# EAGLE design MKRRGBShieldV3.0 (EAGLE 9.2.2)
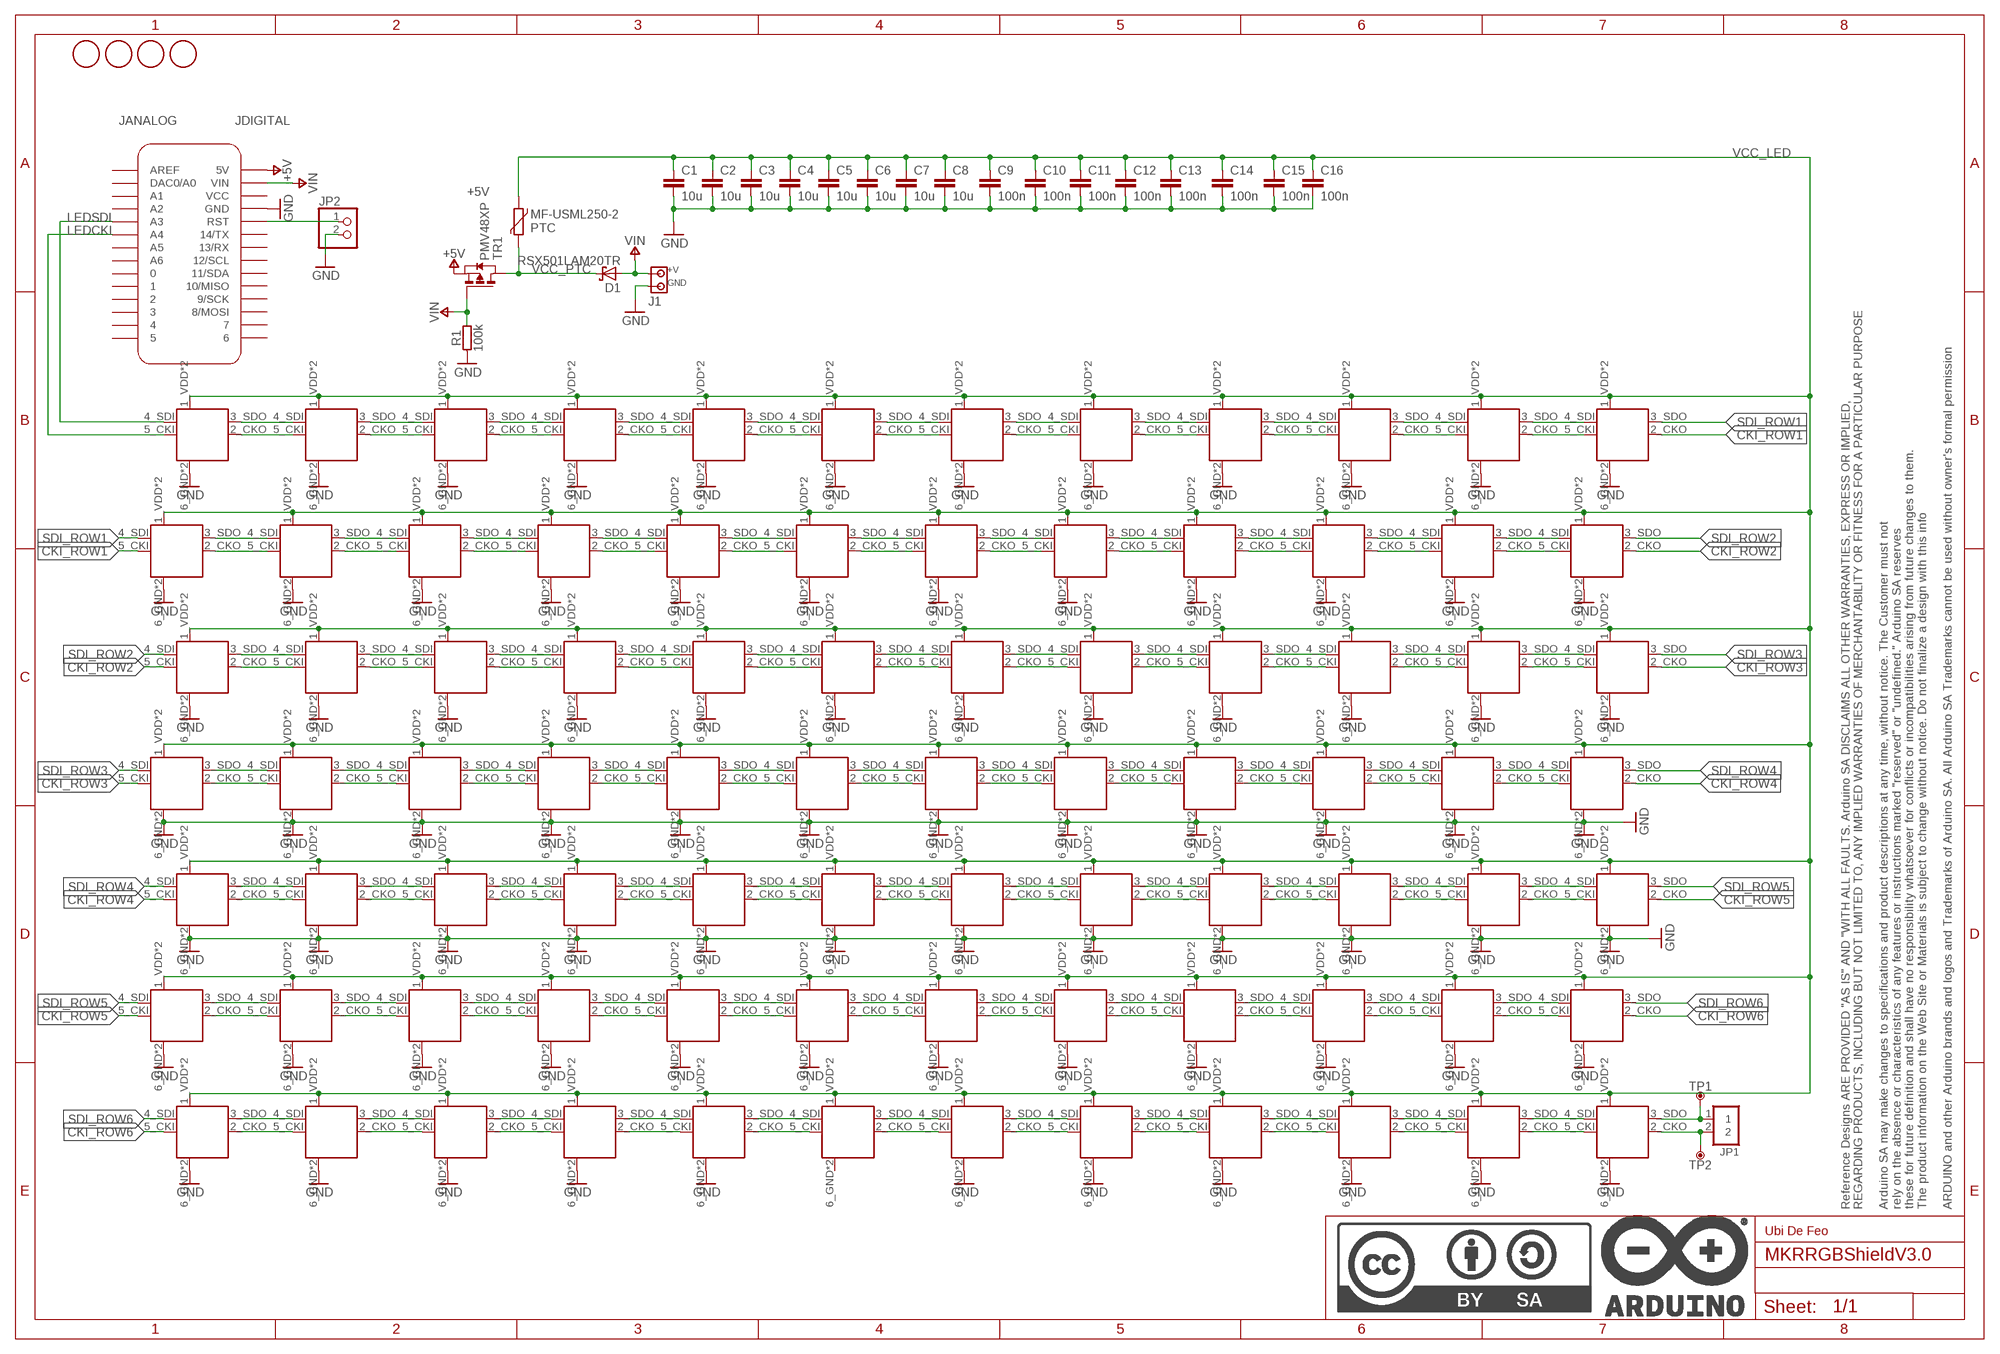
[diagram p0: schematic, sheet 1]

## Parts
32  APA1022020-2018  [APA102-2020_2018]
70  APA1022020-2018  [APA102-2020_2018]
C1  10u  C-10UF-0603  [0603-1608X90N]
C2  10u  C-10UF-0603  [0603-1608X90N]
C3  10u  C-10UF-0603  [0603-1608X90N]
C4  10u  C-10UF-0603  [0603-1608X90N]
C5  10u  C-10UF-0603  [0603-1608X90N]
C6  10u  C-10UF-0603  [0603-1608X90N]
C7  10u  C-10UF-0603  [0603-1608X90N]
C8  10u  C-10UF-0603  [0603-1608X90N]
C9  100n  C-100NF-0402  [0402-1005X55N]
C10  100n  C-100NF-0402  [0402-1005X55N]
C11  100n  C-100NF-0402  [0402-1005X55N]
C12  100n  C-100NF-0402  [0402-1005X55N]
C13  100n  C-100NF-0402  [0402-1005X55N]
C14  100n  C-100NF-0402  [0402-1005X55N]
C15  100n  C-100NF-0402  [0402-1005X55N]
C16  100n  C-100NF-0402  [0402-1005X55N]
D1  RSX501LAM20TR  D_SCHOTTKY-RSX501-SMA  [SMA_DO214AC]
DL1  APA1022020-2018  [APA102-2020_2018]
DL2  APA1022020-2018  [APA102-2020_2018]
DL3  APA1022020-2018  [APA102-2020_2018]
DL4  APA1022020-2018  [APA102-2020_2018]
DL5  APA1022020-2018  [APA102-2020_2018]
DL6  APA1022020-2018  [APA102-2020_2018]
DL7  APA1022020-2018  [APA102-2020_2018]
DL8  APA1022020-2018  [APA102-2020_2018]
DL9  APA1022020-2018  [APA102-2020_2018]
DL10  APA1022020-2018  [APA102-2020_2018]
DL11  APA1022020-2018  [APA102-2020_2018]
DL12  APA1022020-2018  [APA102-2020_2018]
DL13  APA1022020-2018  [APA102-2020_2018]
DL14  APA1022020-2018  [APA102-2020_2018]
DL15  APA1022020-2018  [APA102-2020_2018]
DL16  APA1022020-2018  [APA102-2020_2018]
DL17  APA1022020-2018  [APA102-2020_2018]
DL18  APA1022020-2018  [APA102-2020_2018]
DL19  APA1022020-2018  [APA102-2020_2018]
DL20  APA1022020-2018  [APA102-2020_2018]
DL21  APA1022020-2018  [APA102-2020_2018]
DL22  APA1022020-2018  [APA102-2020_2018]
DL23  APA1022020-2018  [APA102-2020_2018]
DL24  APA1022020-2018  [APA102-2020_2018]
DL25  APA1022020-2018  [APA102-2020_2018]
DL26  APA1022020-2018  [APA102-2020_2018]
DL28  APA1022020-2018  [APA102-2020_2018]
DL29  APA1022020-2018  [APA102-2020_2018]
DL30  APA1022020-2018  [APA102-2020_2018]
DL31  APA1022020-2018  [APA102-2020_2018]
DL33  APA1022020-2018  [APA102-2020_2018]
DL34  APA1022020-2018  [APA102-2020_2018]
DL35  APA1022020-2018  [APA102-2020_2018]
DL36  APA1022020-2018  [APA102-2020_2018]
DL37  APA1022020-2018  [APA102-2020_2018]
DL38  APA1022020-2018  [APA102-2020_2018]
DL39  APA1022020-2018  [APA102-2020_2018]
DL40  APA1022020-2018  [APA102-2020_2018]
DL41  APA1022020-2018  [APA102-2020_2018]
DL42  APA1022020-2018  [APA102-2020_2018]
DL43  APA1022020-2018  [APA102-2020_2018]
DL44  APA1022020-2018  [APA102-2020_2018]
DL45  APA1022020-2018  [APA102-2020_2018]
DL46  APA1022020-2018  [APA102-2020_2018]
DL47  APA1022020-2018  [APA102-2020_2018]
DL48  APA1022020-2018  [APA102-2020_2018]
DL49  APA1022020-2018  [APA102-2020_2018]
DL50  APA1022020-2018  [APA102-2020_2018]
DL51  APA1022020-2018  [APA102-2020_2018]
DL52  APA1022020-2018  [APA102-2020_2018]
DL53  APA1022020-2018  [APA102-2020_2018]
DL54  APA1022020-2018  [APA102-2020_2018]
DL55  APA1022020-2018  [APA102-2020_2018]
DL56  APA1022020-2018  [APA102-2020_2018]
DL57  APA1022020-2018  [APA102-2020_2018]
DL58  APA1022020-2018  [APA102-2020_2018]
DL59  APA1022020-2018  [APA102-2020_2018]
DL60  APA1022020-2018  [APA102-2020_2018]
DL61  APA1022020-2018  [APA102-2020_2018]
DL62  APA1022020-2018  [APA102-2020_2018]
DL63  APA1022020-2018  [APA102-2020_2018]
DL64  APA1022020-2018  [APA102-2020_2018]
DL65  APA1022020-2018  [APA102-2020_2018]
DL66  APA1022020-2018  [APA102-2020_2018]
DL67  APA1022020-2018  [APA102-2020_2018]
DL68  APA1022020-2018  [APA102-2020_2018]
DL69  APA1022020-2018  [APA102-2020_2018]
DL71  APA1022020-2018  [APA102-2020_2018]
DL72  APA1022020-2018  [APA102-2020_2018]
DL73  APA1022020-2018  [APA102-2020_2018]
DL74  APA1022020-2018  [APA102-2020_2018]
DL75  APA1022020-2018  [APA102-2020_2018]
DL76  APA1022020-2018  [APA102-2020_2018]
DL77  APA1022020-2018  [APA102-2020_2018]
DL78  APA1022020-2018  [APA102-2020_2018]
DL79  APA1022020-2018  [APA102-2020_2018]
DL80  APA1022020-2018  [APA102-2020_2018]
DL81  APA1022020-2018  [APA102-2020_2018]
DL82  APA1022020-2018  [APA102-2020_2018]
DL83  APA1022020-2018  [APA102-2020_2018]
DL84  APA1022020-2018  [APA102-2020_2018]
FD1  DNP  FIDUCIAL-1.5MM  [FD-1-1.5]
FD2  DNP  FIDUCIAL-1.5MM  [FD-1-1.5]
FD3  DNP  FIDUCIAL-1.5MM  [FD-1-1.5]
FD4  DNP  FIDUCIAL-1.5MM  [FD-1-1.5]
FRAME1  DNP  A3-FRAME  [FRAME]
J1  -  SCREW2X2.54  [SCREW2]
JANALOG  -  PINHD-1X14-SMD-MKRRGB  [PINHD-DUMMY-1X14-MKRRGB]
JDIGITAL  -  PINHD-1X14-SMD-MKRRGB  [PINHD-DUMMY-1X14-MKRRGB]
JP1  1X02  [1X02]
JP2  PINHD-1X2  [1X02]
MKR1  DNP  MKRBOARD-SMDPIN  [MKRBOARD-SMD-PIN]
PTC  MF-USML250-2  PPTC-MF-USML250-2  [PPTC-1210]
R1  100k  R-100K-0402  [0402-1005X55N]
TP1  DNP  TPTP-1.27MM  [TP-1.27MM]
TP2  DNP  TPTP-1.27MM  [TP-1.27MM]
TR1  PMV48XP  [SOT-23]
U$29  APA1022020-2018  [APA102-2020_2018]

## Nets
+5V: MKR1.5V TR1.2(S)
CKI_ROW1: DL12.2_CKO(CKO) DL13.5_CKI(CKI)
CKI_ROW2: DL24.2_CKO(CKO) DL25.5_CKI(CKI)
CKI_ROW3: DL36.2_CKO(CKO) DL37.5_CKI(CKI)
CKI_ROW4: DL48.2_CKO(CKO) DL49.5_CKI(CKI)
CKI_ROW5: DL60.2_CKO(CKO) DL61.5_CKI(CKI)
CKI_ROW6: DL72.2_CKO(CKO) DL73.5_CKI(CKI)
CKO: DL84.2_CKO(CKO) JP1.2 TP2.X
CKO0: DL1.2_CKO(CKO) DL2.5_CKI(CKI)
DL27: DL28.5_CKI(CKI) U$29.2_CKO(CKO)
GND: 32.6_GND(GND) 32.GNDPAD(GND) 70.6_GND(GND) 70.GNDPAD(GND) C1.2 C2.2 C3.2 C4.2 C5.2 C6.2 C7.2 C8.2 C9.2 C10.2 C11.2 C12.2 C13.2 C14.2 C15.2 C16.2 DL1.6_GND(GND) DL1.GNDPAD(GND) DL2.6_GND(GND) DL2.GNDPAD(GND) DL3.6_GND(GND) DL3.GNDPAD(GND) DL4.6_GND(GND) DL4.GNDPAD(GND) DL5.6_GND(GND) DL5.GNDPAD(GND) DL6.6_GND(GND) DL6.GNDPAD(GND) DL7.6_GND(GND) DL7.GNDPAD(GND) DL8.6_GND(GND) DL8.GNDPAD(GND) DL9.6_GND(GND) DL9.GNDPAD(GND) DL10.6_GND(GND) DL10.GNDPAD(GND) DL11.6_GND(GND) DL11.GNDPAD(GND) DL12.6_GND(GND) DL12.GNDPAD(GND) DL13.6_GND(GND) DL13.GNDPAD(GND) DL14.6_GND(GND) DL14.GNDPAD(GND) DL15.6_GND(GND) DL15.GNDPAD(GND) DL16.6_GND(GND) DL16.GNDPAD(GND) DL17.6_GND(GND) DL17.GNDPAD(GND) DL18.6_GND(GND) DL18.GNDPAD(GND) DL19.6_GND(GND) DL19.GNDPAD(GND) DL20.6_GND(GND) DL20.GNDPAD(GND) DL21.6_GND(GND) DL21.GNDPAD(GND) DL22.6_GND(GND) DL22.GNDPAD(GND) DL23.6_GND(GND) DL23.GNDPAD(GND) DL24.6_GND(GND) DL24.GNDPAD(GND) DL25.6_GND(GND) DL25.GNDPAD(GND) DL26.6_GND(GND) DL26.GNDPAD(GND) DL28.6_GND(GND) DL28.GNDPAD(GND) DL29.6_GND(GND) DL29.GNDPAD(GND) DL30.6_GND(GND) DL30.GNDPAD(GND) DL31.6_GND(GND) DL31.GNDPAD(GND) DL33.6_GND(GND) DL33.GNDPAD(GND) DL34.6_GND(GND) DL34.GNDPAD(GND) DL35.6_GND(GND) DL35.GNDPAD(GND) DL36.6_GND(GND) DL36.GNDPAD(GND) DL37.6_GND(GND) DL37.GNDPAD(GND) DL38.6_GND(GND) DL38.GNDPAD(GND) DL39.6_GND(GND) DL39.GNDPAD(GND) DL40.6_GND(GND) DL40.GNDPAD(GND) DL41.6_GND(GND) DL41.GNDPAD(GND) DL42.6_GND(GND) DL42.GNDPAD(GND) DL43.6_GND(GND) DL43.GNDPAD(GND) DL44.6_GND(GND) DL44.GNDPAD(GND) DL45.6_GND(GND) DL45.GNDPAD(GND) DL46.6_GND(GND) DL46.GNDPAD(GND) DL47.6_GND(GND) DL47.GNDPAD(GND) DL48.6_GND(GND) DL48.GNDPAD(GND) DL49.6_GND(GND) DL49.GNDPAD(GND) DL50.6_GND(GND) DL50.GNDPAD(GND) DL51.6_GND(GND) DL51.GNDPAD(GND) DL52.6_GND(GND) DL52.GNDPAD(GND) DL53.6_GND(GND) DL53.GNDPAD(GND) DL54.6_GND(GND) DL54.GNDPAD(GND) DL55.6_GND(GND) DL55.GNDPAD(GND) DL56.6_GND(GND) DL56.GNDPAD(GND) DL57.6_GND(GND) DL57.GNDPAD(GND) DL58.6_GND(GND) DL58.GNDPAD(GND) DL59.6_GND(GND) DL59.GNDPAD(GND) DL60.6_GND(GND) DL60.GNDPAD(GND) DL61.6_GND(GND) DL61.GNDPAD(GND) DL62.6_GND(GND) DL62.GNDPAD(GND) DL63.6_GND(GND) DL63.GNDPAD(GND) DL64.6_GND(GND) DL64.GNDPAD(GND) DL65.6_GND(GND) DL65.GNDPAD(GND) DL66.6_GND(GND) DL66.GNDPAD(GND) DL67.6_GND(GND) DL67.GNDPAD(GND) DL68.6_GND(GND) DL68.GNDPAD(GND) DL69.6_GND(GND) DL69.GNDPAD(GND) DL71.6_GND(GND) DL71.GNDPAD(GND) DL72.6_GND(GND) DL72.GNDPAD(GND) DL73.6_GND(GND) DL73.GNDPAD(GND) DL74.6_GND(GND) DL74.GNDPAD(GND) DL75.6_GND(GND) DL75.GNDPAD(GND) DL76.6_GND(GND) DL76.GNDPAD(GND) DL77.6_GND(GND) DL77.GNDPAD(GND) DL79.6_GND(GND) DL79.GNDPAD(GND) DL80.6_GND(GND) DL80.GNDPAD(GND) DL81.6_GND(GND) DL81.GNDPAD(GND) DL82.6_GND(GND) DL82.GNDPAD(GND) DL83.6_GND(GND) DL83.GNDPAD(GND) DL84.6_GND(GND) DL84.GNDPAD(GND) J1.GND JP2.2 MKR1.GND R1.1 U$29.6_GND(GND) U$29.GNDPAD(GND)
LEDCKI: DL1.5_CKI(CKI) MKR1.A4
LEDSDI: DL1.4_SDI(SDI) MKR1.A3
N$1: DL2.3_SDO(SDO) DL3.4_SDI(SDI)
N$2: DL2.2_CKO(CKO) DL3.5_CKI(CKI)
N$3: DL3.3_SDO(SDO) DL4.4_SDI(SDI)
N$4: DL3.2_CKO(CKO) DL4.5_CKI(CKI)
N$5: DL4.3_SDO(SDO) DL5.4_SDI(SDI)
N$6: DL4.2_CKO(CKO) DL5.5_CKI(CKI)
N$7: DL5.3_SDO(SDO) DL6.4_SDI(SDI)
N$8: DL5.2_CKO(CKO) DL6.5_CKI(CKI)
N$9: DL6.3_SDO(SDO) DL7.4_SDI(SDI)
N$10: DL6.2_CKO(CKO) DL7.5_CKI(CKI)
N$11: DL7.3_SDO(SDO) DL8.4_SDI(SDI)
N$12: DL7.2_CKO(CKO) DL8.5_CKI(CKI)
N$13: DL8.3_SDO(SDO) DL9.4_SDI(SDI)
N$14: DL8.2_CKO(CKO) DL9.5_CKI(CKI)
N$15: DL9.3_SDO(SDO) DL10.4_SDI(SDI)
N$16: DL9.2_CKO(CKO) DL10.5_CKI(CKI)
N$17: DL10.3_SDO(SDO) DL11.4_SDI(SDI)
N$18: DL10.2_CKO(CKO) DL11.5_CKI(CKI)
N$19: DL11.3_SDO(SDO) DL12.4_SDI(SDI)
N$20: DL11.2_CKO(CKO) DL12.5_CKI(CKI)
N$21: DL13.3_SDO(SDO) DL14.4_SDI(SDI)
N$22: DL13.2_CKO(CKO) DL14.5_CKI(CKI)
N$23: DL14.3_SDO(SDO) DL15.4_SDI(SDI)
N$24: DL14.2_CKO(CKO) DL15.5_CKI(CKI)
N$25: DL15.3_SDO(SDO) DL16.4_SDI(SDI)
N$26: DL15.2_CKO(CKO) DL16.5_CKI(CKI)
N$27: DL16.3_SDO(SDO) DL17.4_SDI(SDI)
N$28: DL16.2_CKO(CKO) DL17.5_CKI(CKI)
N$29: DL17.3_SDO(SDO) DL18.4_SDI(SDI)
N$30: DL17.2_CKO(CKO) DL18.5_CKI(CKI)
N$31: DL18.3_SDO(SDO) DL19.4_SDI(SDI)
N$32: DL18.2_CKO(CKO) DL19.5_CKI(CKI)
N$33: DL19.3_SDO(SDO) DL20.4_SDI(SDI)
N$34: DL19.2_CKO(CKO) DL20.5_CKI(CKI)
N$35: DL20.3_SDO(SDO) DL21.4_SDI(SDI)
N$36: DL20.2_CKO(CKO) DL21.5_CKI(CKI)
N$37: DL21.3_SDO(SDO) DL22.4_SDI(SDI)
N$38: DL21.2_CKO(CKO) DL22.5_CKI(CKI)
N$39: DL22.3_SDO(SDO) DL23.4_SDI(SDI)
N$40: DL22.2_CKO(CKO) DL23.5_CKI(CKI)
N$41: DL23.3_SDO(SDO) DL24.4_SDI(SDI)
N$42: DL23.2_CKO(CKO) DL24.5_CKI(CKI)
N$43: DL25.3_SDO(SDO) DL26.4_SDI(SDI)
N$44: DL25.2_CKO(CKO) DL26.5_CKI(CKI)
N$45: DL26.3_SDO(SDO) U$29.4_SDI(SDI)
N$46: DL26.2_CKO(CKO) U$29.5_CKI(CKI)
N$47: DL28.4_SDI(SDI) U$29.3_SDO(SDO)
N$49: DL28.3_SDO(SDO) DL29.4_SDI(SDI)
N$50: DL28.2_CKO(CKO) DL29.5_CKI(CKI)
N$51: DL29.3_SDO(SDO) DL30.4_SDI(SDI)
N$52: DL29.2_CKO(CKO) DL30.5_CKI(CKI)
N$53: DL30.3_SDO(SDO) DL31.4_SDI(SDI)
N$54: DL30.2_CKO(CKO) DL31.5_CKI(CKI)
N$55: 32.4_SDI(SDI) DL31.3_SDO(SDO)
N$56: 32.5_CKI(CKI) DL31.2_CKO(CKO)
N$57: 32.3_SDO(SDO) DL33.4_SDI(SDI)
N$58: 32.2_CKO(CKO) DL33.5_CKI(CKI)
N$59: DL33.3_SDO(SDO) DL34.4_SDI(SDI)
N$60: DL33.2_CKO(CKO) DL34.5_CKI(CKI)
N$61: DL34.3_SDO(SDO) DL35.4_SDI(SDI)
N$62: DL34.2_CKO(CKO) DL35.5_CKI(CKI)
N$63: DL35.3_SDO(SDO) DL36.4_SDI(SDI)
N$64: DL35.2_CKO(CKO) DL36.5_CKI(CKI)
N$65: DL37.3_SDO(SDO) DL38.4_SDI(SDI)
N$66: DL37.2_CKO(CKO) DL38.5_CKI(CKI)
N$67: DL38.3_SDO(SDO) DL39.4_SDI(SDI)
N$68: DL38.2_CKO(CKO) DL39.5_CKI(CKI)
N$69: DL39.3_SDO(SDO) DL40.4_SDI(SDI)
N$70: DL39.2_CKO(CKO) DL40.5_CKI(CKI)
N$71: DL40.3_SDO(SDO) DL41.4_SDI(SDI)
N$72: DL40.2_CKO(CKO) DL41.5_CKI(CKI)
N$73: DL41.3_SDO(SDO) DL42.4_SDI(SDI)
N$74: DL41.2_CKO(CKO) DL42.5_CKI(CKI)
N$75: DL42.3_SDO(SDO) DL43.4_SDI(SDI)
N$76: DL42.2_CKO(CKO) DL43.5_CKI(CKI)
N$77: DL43.3_SDO(SDO) DL44.4_SDI(SDI)
N$78: DL43.2_CKO(CKO) DL44.5_CKI(CKI)
N$79: DL44.3_SDO(SDO) DL45.4_SDI(SDI)
N$80: DL44.2_CKO(CKO) DL45.5_CKI(CKI)
N$81: DL45.3_SDO(SDO) DL46.4_SDI(SDI)
N$82: DL45.2_CKO(CKO) DL46.5_CKI(CKI)
N$83: DL46.3_SDO(SDO) DL47.4_SDI(SDI)
N$84: DL46.2_CKO(CKO) DL47.5_CKI(CKI)
N$85: DL47.3_SDO(SDO) DL48.4_SDI(SDI)
N$86: DL47.2_CKO(CKO) DL48.5_CKI(CKI)
N$87: DL50.3_SDO(SDO) DL51.4_SDI(SDI)
N$88: DL50.2_CKO(CKO) DL51.5_CKI(CKI)
N$89: DL51.3_SDO(SDO) DL52.4_SDI(SDI)
N$90: DL51.2_CKO(CKO) DL52.5_CKI(CKI)
N$91: DL52.3_SDO(SDO) DL53.4_SDI(SDI)
N$92: DL52.2_CKO(CKO) DL53.5_CKI(CKI)
N$93: DL53.3_SDO(SDO) DL54.4_SDI(SDI)
N$94: DL53.2_CKO(CKO) DL54.5_CKI(CKI)
N$95: DL54.3_SDO(SDO) DL55.4_SDI(SDI)
N$96: DL54.2_CKO(CKO) DL55.5_CKI(CKI)
N$97: DL55.3_SDO(SDO) DL56.4_SDI(SDI)
N$98: DL55.2_CKO(CKO) DL56.5_CKI(CKI)
N$99: DL56.3_SDO(SDO) DL57.4_SDI(SDI)
N$100: DL56.2_CKO(CKO) DL57.5_CKI(CKI)
N$101: DL57.3_SDO(SDO) DL58.4_SDI(SDI)
N$102: DL57.2_CKO(CKO) DL58.5_CKI(CKI)
N$103: DL58.3_SDO(SDO) DL59.4_SDI(SDI)
N$104: DL58.2_CKO(CKO) DL59.5_CKI(CKI)
N$105: DL59.3_SDO(SDO) DL60.4_SDI(SDI)
N$106: DL59.2_CKO(CKO) DL60.5_CKI(CKI)
N$107: DL49.3_SDO(SDO) DL50.4_SDI(SDI)
N$108: DL49.2_CKO(CKO) DL50.5_CKI(CKI)
N$109: DL61.3_SDO(SDO) DL62.4_SDI(SDI)
N$110: DL61.2_CKO(CKO) DL62.5_CKI(CKI)
N$111: DL62.3_SDO(SDO) DL63.4_SDI(SDI)
N$112: DL62.2_CKO(CKO) DL63.5_CKI(CKI)
N$113: DL73.3_SDO(SDO) DL74.4_SDI(SDI)
N$114: DL73.2_CKO(CKO) DL74.5_CKI(CKI)
N$115: DL74.3_SDO(SDO) DL75.4_SDI(SDI)
N$116: DL74.2_CKO(CKO) DL75.5_CKI(CKI)
N$117: DL63.3_SDO(SDO) DL64.4_SDI(SDI)
N$118: DL63.2_CKO(CKO) DL64.5_CKI(CKI)
N$119: DL75.3_SDO(SDO) DL76.4_SDI(SDI)
N$120: DL75.2_CKO(CKO) DL76.5_CKI(CKI)
N$121: DL64.3_SDO(SDO) DL65.4_SDI(SDI)
N$122: DL64.2_CKO(CKO) DL65.5_CKI(CKI)
N$123: DL76.3_SDO(SDO) DL77.4_SDI(SDI)
N$124: DL76.2_CKO(CKO) DL77.5_CKI(CKI)
N$125: DL65.3_SDO(SDO) DL66.4_SDI(SDI)
N$126: DL65.2_CKO(CKO) DL66.5_CKI(CKI)
N$127: DL77.3_SDO(SDO) DL78.4_SDI(SDI)
N$128: DL77.2_CKO(CKO) DL78.5_CKI(CKI)
N$129: DL66.3_SDO(SDO) DL67.4_SDI(SDI)
N$130: DL66.2_CKO(CKO) DL67.5_CKI(CKI)
N$131: DL78.3_SDO(SDO) DL79.4_SDI(SDI)
N$132: DL78.2_CKO(CKO) DL79.5_CKI(CKI)
N$133: DL67.3_SDO(SDO) DL68.4_SDI(SDI)
N$134: DL67.2_CKO(CKO) DL68.5_CKI(CKI)
N$135: DL79.3_SDO(SDO) DL80.4_SDI(SDI)
N$136: DL79.2_CKO(CKO) DL80.5_CKI(CKI)
N$137: DL68.3_SDO(SDO) DL69.4_SDI(SDI)
N$138: DL68.2_CKO(CKO) DL69.5_CKI(CKI)
N$139: DL80.3_SDO(SDO) DL81.4_SDI(SDI)
N$140: DL80.2_CKO(CKO) DL81.5_CKI(CKI)
N$141: 70.4_SDI(SDI) DL69.3_SDO(SDO)
N$142: 70.5_CKI(CKI) DL69.2_CKO(CKO)
N$143: DL81.3_SDO(SDO) DL82.4_SDI(SDI)
N$144: DL81.2_CKO(CKO) DL82.5_CKI(CKI)
N$145: 70.3_SDO(SDO) DL71.4_SDI(SDI)
N$146: 70.2_CKO(CKO) DL71.5_CKI(CKI)
N$147: DL82.3_SDO(SDO) DL83.4_SDI(SDI)
N$148: DL82.2_CKO(CKO) DL83.5_CKI(CKI)
N$149: DL71.3_SDO(SDO) DL72.4_SDI(SDI)
N$150: DL71.2_CKO(CKO) DL72.5_CKI(CKI)
N$151: DL83.3_SDO(SDO) DL84.4_SDI(SDI)
N$152: DL83.2_CKO(CKO) DL84.5_CKI(CKI)
RESET: JP2.1 MKR1.RST
SDI_ROW1: DL12.3_SDO(SDO) DL13.4_SDI(SDI)
SDI_ROW2: DL24.3_SDO(SDO) DL25.4_SDI(SDI)
SDI_ROW3: DL36.3_SDO(SDO) DL37.4_SDI(SDI)
SDI_ROW4: DL48.3_SDO(SDO) DL49.4_SDI(SDI)
SDI_ROW5: DL60.3_SDO(SDO) DL61.4_SDI(SDI)
SDI_ROW6: DL72.3_SDO(SDO) DL73.4_SDI(SDI)
SDO: DL84.3_SDO(SDO) JP1.1 TP1.X
SDO0: DL1.3_SDO(SDO) DL2.4_SDI(SDI)
VCC_LED: 32.1_VDD(VCC) 32.VDDPAD(VCC) 70.1_VDD(VCC) 70.VDDPAD(VCC) C1.1 C2.1 C3.1 C4.1 C5.1 C6.1 C7.1 C8.1 C9.1 C10.1 C11.1 C12.1 C13.1 C14.1 C15.1 C16.1 DL1.1_VDD(VCC) DL1.VDDPAD(VCC) DL2.1_VDD(VCC) DL2.VDDPAD(VCC) DL3.1_VDD(VCC) DL3.VDDPAD(VCC) DL4.1_VDD(VCC) DL4.VDDPAD(VCC) DL5.1_VDD(VCC) DL5.VDDPAD(VCC) DL6.1_VDD(VCC) DL6.VDDPAD(VCC) DL7.1_VDD(VCC) DL7.VDDPAD(VCC) DL8.1_VDD(VCC) DL8.VDDPAD(VCC) DL9.1_VDD(VCC) DL9.VDDPAD(VCC) DL10.1_VDD(VCC) DL10.VDDPAD(VCC) DL11.1_VDD(VCC) DL11.VDDPAD(VCC) DL12.1_VDD(VCC) DL12.VDDPAD(VCC) DL13.1_VDD(VCC) DL13.VDDPAD(VCC) DL14.1_VDD(VCC) DL14.VDDPAD(VCC) DL15.1_VDD(VCC) DL15.VDDPAD(VCC) DL16.1_VDD(VCC) DL16.VDDPAD(VCC) DL17.1_VDD(VCC) DL17.VDDPAD(VCC) DL18.1_VDD(VCC) DL18.VDDPAD(VCC) DL19.1_VDD(VCC) DL19.VDDPAD(VCC) DL20.1_VDD(VCC) DL20.VDDPAD(VCC) DL21.1_VDD(VCC) DL21.VDDPAD(VCC) DL22.1_VDD(VCC) DL22.VDDPAD(VCC) DL23.1_VDD(VCC) DL23.VDDPAD(VCC) DL24.1_VDD(VCC) DL24.VDDPAD(VCC) DL25.1_VDD(VCC) DL25.VDDPAD(VCC) DL26.1_VDD(VCC) DL26.VDDPAD(VCC) DL28.1_VDD(VCC) DL28.VDDPAD(VCC) DL29.1_VDD(VCC) DL29.VDDPAD(VCC) DL30.1_VDD(VCC) DL30.VDDPAD(VCC) DL31.1_VDD(VCC) DL31.VDDPAD(VCC) DL33.1_VDD(VCC) DL33.VDDPAD(VCC) DL34.1_VDD(VCC) DL34.VDDPAD(VCC) DL35.1_VDD(VCC) DL35.VDDPAD(VCC) DL36.1_VDD(VCC) DL36.VDDPAD(VCC) DL37.1_VDD(VCC) DL37.VDDPAD(VCC) DL38.1_VDD(VCC) DL38.VDDPAD(VCC) DL39.1_VDD(VCC) DL39.VDDPAD(VCC) DL40.1_VDD(VCC) DL40.VDDPAD(VCC) DL41.1_VDD(VCC) DL41.VDDPAD(VCC) DL42.1_VDD(VCC) DL42.VDDPAD(VCC) DL43.1_VDD(VCC) DL43.VDDPAD(VCC) DL44.1_VDD(VCC) DL44.VDDPAD(VCC) DL45.1_VDD(VCC) DL45.VDDPAD(VCC) DL46.1_VDD(VCC) DL46.VDDPAD(VCC) DL47.1_VDD(VCC) DL47.VDDPAD(VCC) DL48.1_VDD(VCC) DL48.VDDPAD(VCC) DL49.1_VDD(VCC) DL49.VDDPAD(VCC) DL50.1_VDD(VCC) DL50.VDDPAD(VCC) DL51.1_VDD(VCC) DL51.VDDPAD(VCC) DL52.1_VDD(VCC) DL52.VDDPAD(VCC) DL53.1_VDD(VCC) DL53.VDDPAD(VCC) DL54.1_VDD(VCC) DL54.VDDPAD(VCC) DL55.1_VDD(VCC) DL55.VDDPAD(VCC) DL56.1_VDD(VCC) DL56.VDDPAD(VCC) DL57.1_VDD(VCC) DL57.VDDPAD(VCC) DL58.1_VDD(VCC) DL58.VDDPAD(VCC) DL59.1_VDD(VCC) DL59.VDDPAD(VCC) DL60.1_VDD(VCC) DL60.VDDPAD(VCC) DL61.1_VDD(VCC) DL61.VDDPAD(VCC) DL62.1_VDD(VCC) DL62.VDDPAD(VCC) DL63.1_VDD(VCC) DL63.VDDPAD(VCC) DL64.1_VDD(VCC) DL64.VDDPAD(VCC) DL65.1_VDD(VCC) DL65.VDDPAD(VCC) DL66.1_VDD(VCC) DL66.VDDPAD(VCC) DL67.1_VDD(VCC) DL67.VDDPAD(VCC) DL68.1_VDD(VCC) DL68.VDDPAD(VCC) DL69.1_VDD(VCC) DL69.VDDPAD(VCC) DL71.1_VDD(VCC) DL71.VDDPAD(VCC) DL72.1_VDD(VCC) DL72.VDDPAD(VCC) DL73.1_VDD(VCC) DL73.VDDPAD(VCC) DL74.1_VDD(VCC) DL74.VDDPAD(VCC) DL75.1_VDD(VCC) DL75.VDDPAD(VCC) DL76.1_VDD(VCC) DL76.VDDPAD(VCC) DL77.1_VDD(VCC) DL77.VDDPAD(VCC) DL78.1_VDD(VCC) DL78.VDDPAD(VCC) DL79.1_VDD(VCC) DL79.VDDPAD(VCC) DL80.1_VDD(VCC) DL80.VDDPAD(VCC) DL81.1_VDD(VCC) DL81.VDDPAD(VCC) DL82.1_VDD(VCC) DL82.VDDPAD(VCC) DL83.1_VDD(VCC) DL83.VDDPAD(VCC) DL84.1_VDD(VCC) DL84.VDDPAD(VCC) PTC.P$1 U$29.1_VDD(VCC) U$29.VDDPAD(VCC)
VCC_PTC: D1.C PTC.P$2 TR1.1(D)
VIN: D1.A J1.V+ MKR1.VIN R1.2 TR1.3(G)
Unconnected: MKR1.0 MKR1.1 MKR1.2 MKR1.3 MKR1.4 MKR1.5 MKR1.6 MKR1.7 MKR1.8(8/MOSI) MKR1.9(9/SCK) MKR1.10(10/MISO) MKR1.11(11/SDA) MKR1.12(12/SCL) MKR1.13(13/RX) MKR1.14(14/TX) MKR1.A1 MKR1.A2 MKR1.A5 MKR1.A6 MKR1.AREF MKR1.DAC0/A0 MKR1.VCC

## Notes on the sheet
- Ubi De Feo

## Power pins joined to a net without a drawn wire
GND: DL78.6_GND(GND) DL78.GNDPAD(GND)

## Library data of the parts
32 70 DL1-DL26 DL28-DL31 DL33-DL69 DL71-DL84 U$29 = Arduino-diodes:APA102: -; CODE-ARDUINO: A5307
C1-C8 = Arduino-rcl:C: SMD Capacitor; CODE-ARDUINO: 2213; DATASHEET: http://www.murata.com/~/media/webrenewal/support/library/catalog/products/capacitor/mlcc/c02e.pdf; DISTRIBUTOR-LINK: http://www.digikey.com/product-search/en?keywords=490-10728-1-ND; DISTRIBUTOR-PN: 490-10728-1-ND; MANUFACTURER: Murata; MANUFACTURER-PN: GRM188R61C106KAALD; NOTE: -
C9-C16 = Arduino-rcl:C: SMD Capacitor; CODE-ARDUINO: 0132; DATASHEET: http://www.tdk.com/pdf/TDKMLCCCapRange.pdf; DISTRIBUTOR-LINK: http://www.digikey.com/product-detail/en/tdk-corporation/C1005X5R1H104K050BB/445-5942-1-ND/2443982; DISTRIBUTOR-PN: 445-5942-1-ND; MANUFACTURER: TDK; MANUFACTURER-PN: C1005X5R1H104K050BB; NOTE: -
D1 = Arduino-diodes:D_SCHOTTKY: Schottky Diodes; CODE-ARDUINO: A5388; DATASHEET: https://www.rohm.com/datasheet/RSX501LAM20/rsx501lam20tr-e; DISTRIBUTOR-LINK: https://www.digikey.com/product-detail/en/rohm-semiconductor/RSX501LAM20TR/RSX501LAM20TR-ND/7318348; DISTRIBUTOR-PN: RSX501LAM20TR-ND; MANUFACTURER: Rohm; MANUFACTURER-PN: RSX501LAM20TR
FD1-FD4 = Arduino-utility:FIDUCIAL: Fiducial mount; CODE-ARDUINO: DNP; DATASHEET: DNP; DISTRIBUTOR-LINK: DNP; DISTRIBUTOR-PN: DNP; MANUFACTURER: DNP; MANUFACTURER-PN: DNP
FRAME1 = Arduino-utility:A3-FRAME; CODE-ARDUINO: DNP; DATASHEET: DNP; DISTRIBUTOR-LINK: DNP; DISTRIBUTOR-PN: DNP; MANUFACTURER: DNP; MANUFACTURER-PN: DNP; NOTE: DNP
J1 = Arduino-connectors:SCREW2X2.54: 2.45 Screw terminal Block; CODE-ARDUINO: A5401; DATASHEET: http://www.on-shore.com/wp-content/uploads/2015/09/ostvnxxa150.pdf; DISTRIBUTOR-LINK: http://www.digikey.com/product-detail/en/on-shore-technology-inc/OSTVN02A150/ED10561-ND/1588862; DISTRIBUTOR-PN: ED10561-ND; MANUFACTURER: On Shore Technology Inc.; MANUFACTURER-PN: OSTVN02A150
JANALOG JDIGITAL = Arduino-connectors:PINHD-1X14-SMD-MKRRGB: PIN HEADER 1X14 SMD MKRRGB; CODE-ARDUINO: A5476; DATASHEET: -; DISTRIBUTOR-LINK: -; DISTRIBUTOR-PN: -; MANUFACTURER: -; MANUFACTURER-PN: 20TW-489
JP1 = Ai_Connectors:1X02
JP2 = pinhead:PINHD-1X2: PIN HEADER
MKR1 = Arduino-utility:MKRBOARD: MKR board footprint; CODE-ARDUINO: DNP; DATASHEET: DNP; DISTRIBUTOR-LINK: DNP; DISTRIBUTOR-PN: DNP; MANUFACTURER: DNP; MANUFACTURER-PN: DNP
PTC = Arduino-rcl:PPTC-MF-USML250-2: SMD PTC; CODE-ARDUINO: A5352; DATASHEET: https://nl.mouser.com/datasheet/2/54/fusml-1115405.pdf; DISTRIBUTOR-LINK: https://nl.mouser.com/ProductDetail/Bourns/MF-USML250-2?qs=sGAEpiMZZMsgjL4JkW1EEeamwSwzTegDcao9m1Tn2w%252bDqQsyyTArTA==; DISTRIBUTOR-PN: 652-MF-USML250-2; MANUFACTURER: Bourns Inc; MANUFACTURER-PN: MF-USML250-2; NOTE: NO
R1 = Arduino-rcl:R: SMD Resistor; CODE-ARDUINO: 0134; DATASHEET: www.yageo.com.tw/exep/pages/download/literatures/PYu-R_INT-thick_7.pdf; DISTRIBUTOR-LINK: http://www.digikey.com/product-detail/en/yageo/RC0402FR-07100KL/311-100KLRCT-ND/729473; DISTRIBUTOR-PN: 311-100KLRCT-ND; MANUFACTURER: Yageo; MANUFACTURER-PN: RC0402FR-07100KL; NOTE: NO
TP1 TP2 = Arduino-utility:TP: Testpoint; CODE-ARDUINO: DNP; DATASHEET: DNP; DISTRIBUTOR-LINK: DNP; DISTRIBUTOR-PN: DNP; MANUFACTURER: DNP; MANUFACTURER-PN: DNP
TR1 = Arduino-transistors:PMV48XP: 20 V, 3.5 A P-channel Trench MOSFET - PMV48XP; CODE-ARDUINO: 1039; DATASHEET: https://assets.nexperia.com/documents/data-sheet/PMV48XP.pdf; DISTRIBUTOR-LINK: https://www.digikey.com/product-detail/en/nexperia-usa-inc/PMV48XP215/1727-5907-1-ND/2744665; DISTRIBUTOR-PN: 1727-5907-1-ND; MANUFACTURER: Nexperia; MANUFACTURER-PN: PMV48XP,215; PN-ALTERNATIVE: FDN340P; PN-ALTERNATIVE2: IRLML6402TRPBF

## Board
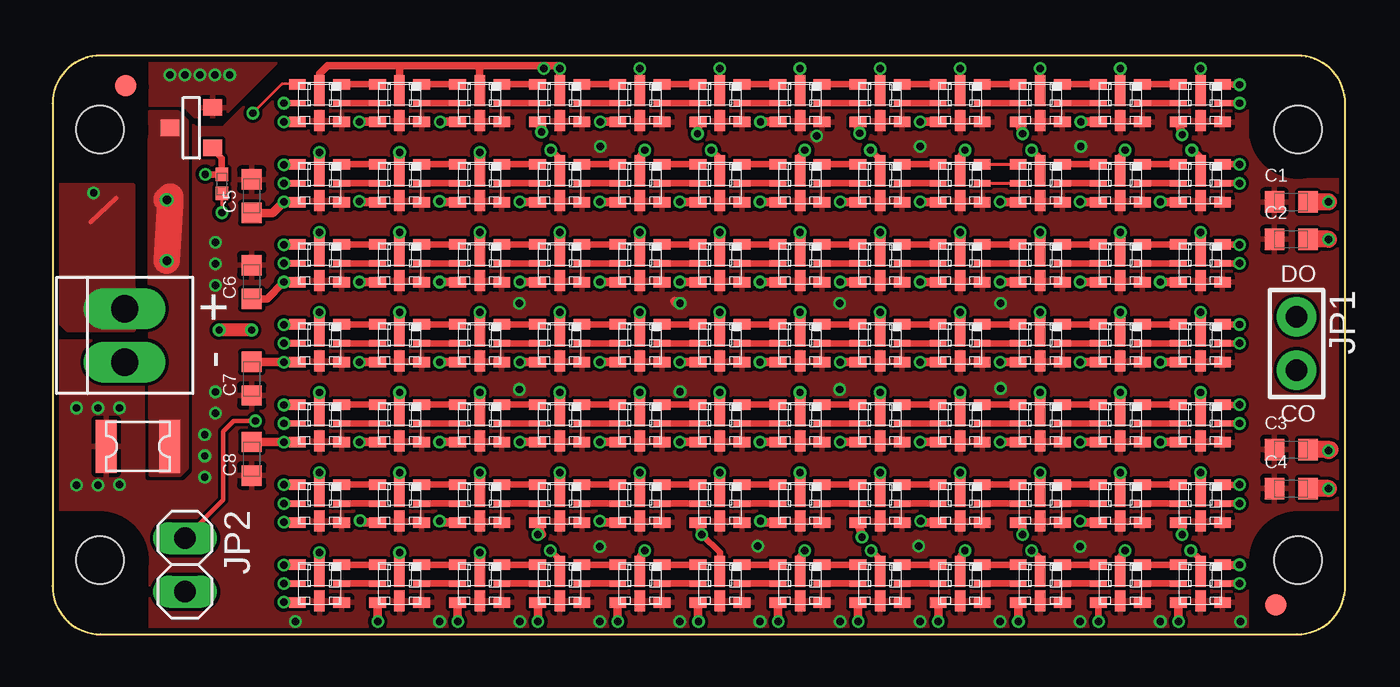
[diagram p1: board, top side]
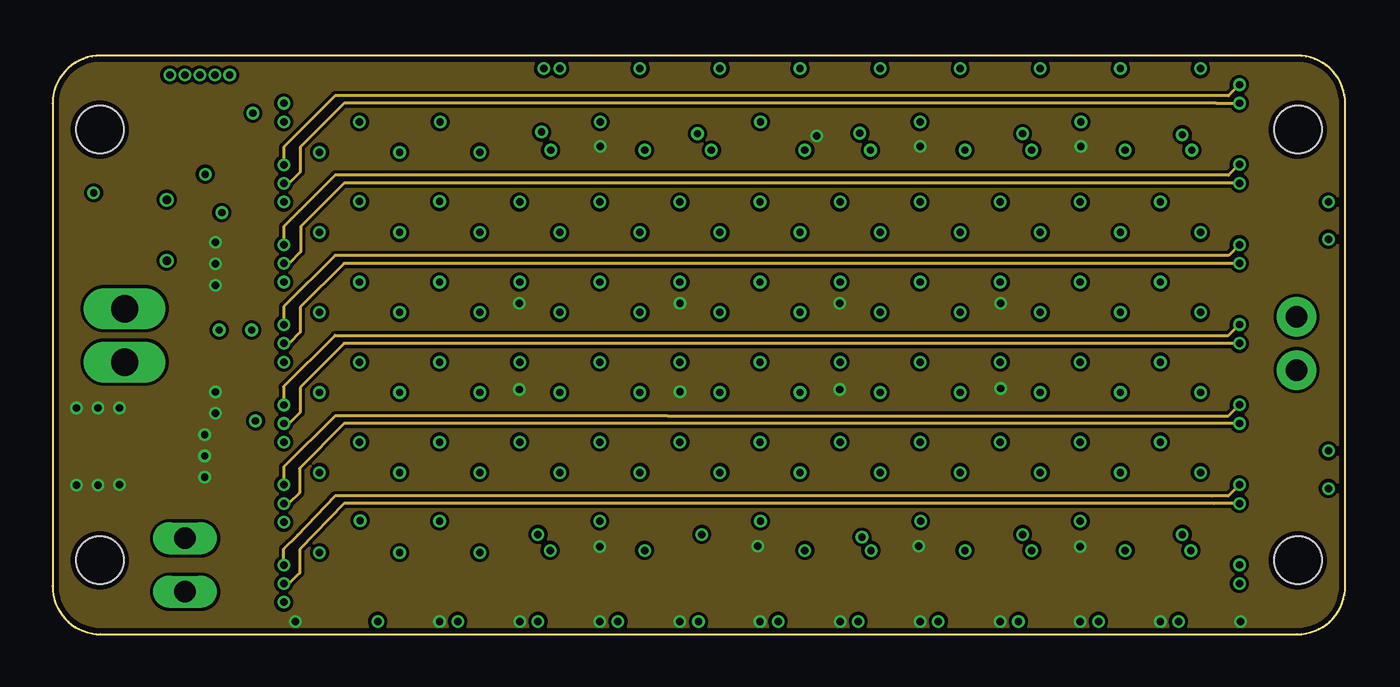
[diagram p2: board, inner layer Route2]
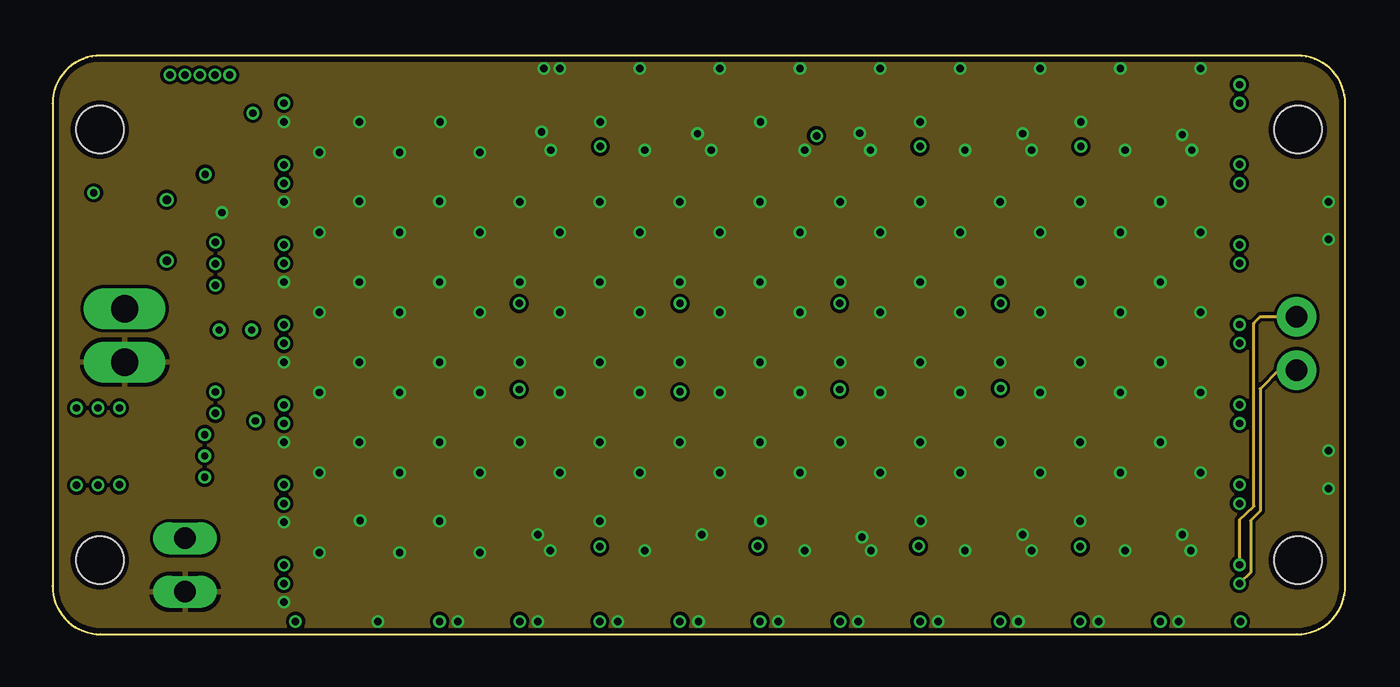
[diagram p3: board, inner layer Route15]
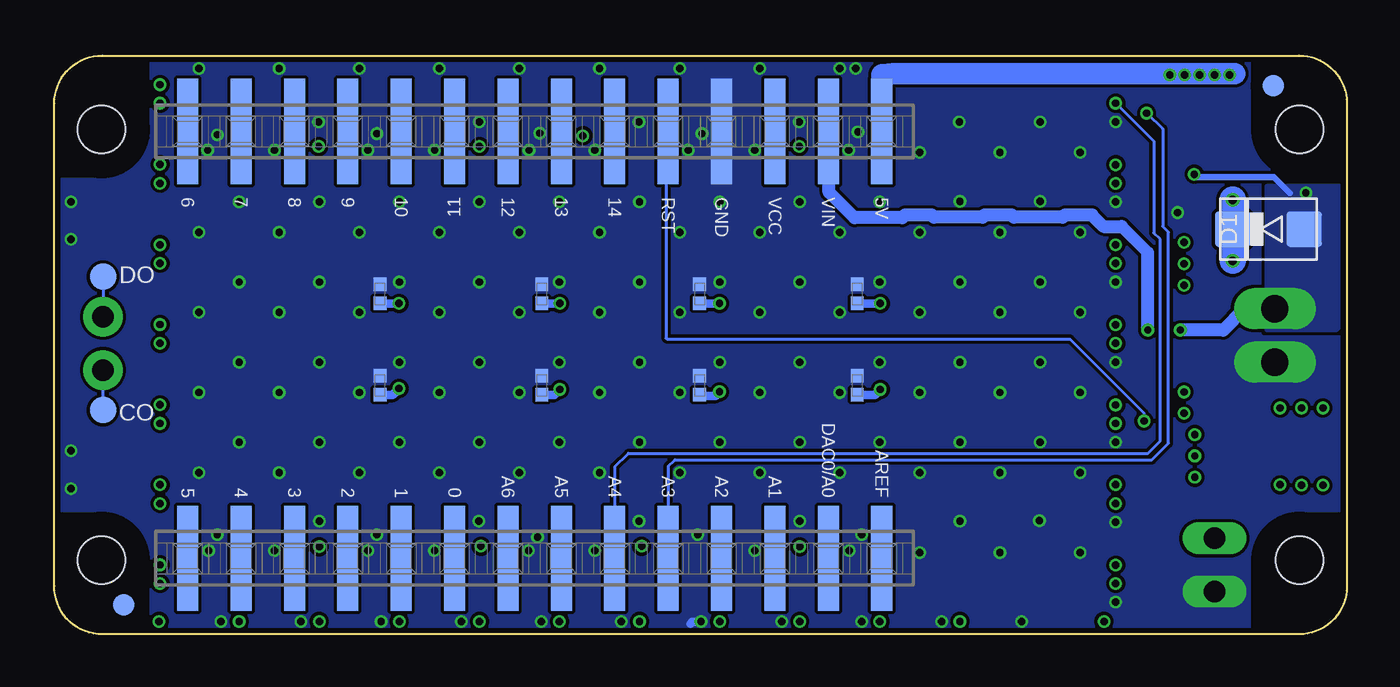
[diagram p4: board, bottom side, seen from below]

Size 61.5 x 27.54 mm. Coordinates in mm from the lower left corner, seen from the top.
Copper layers (1*2*15*16): Top 0.018mm / dielectric 0.36mm / Route2 0.035mm / dielectric 0.71mm / Route15 0.035mm / dielectric 0.2mm / Bottom 0.018mm
Design rules "eC_4Layer_PClass6_BaseCopperO18-I35_eCDefault *": minimum track width 0.15mm, minimum drill 0.35mm, track to track 0.15mm, track to pad 0.15mm, pad to pad 0.15mm, via to via 0.14mm, smd to smd 0mil, copper to edge 0.25mm, drill to drill 0.35mm, minimum pad ring 0.175mm, minimum via ring 0.125mm, stop-mask expansion 0mil, vias tented up to drill 0.45mm, thermal gap 0.2mm

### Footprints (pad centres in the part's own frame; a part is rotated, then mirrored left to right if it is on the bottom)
APA102-2020_2018 = smd 0.8 x 0.5: 1_VDD -1.05,0.9; 3_SDO -1.05,-0.9; 4_SDI 1.05,-0.9; 6_GND 1.05,0.9 | smd 0.8 x 0.3: 2_CKO -1.05,0; 5_CKI 1.05,0 | smd 0.5 x 1.48: GNDPAD 0,-0.59 | smd 0.5 x 1: VDDPAD 0,0.83
0603-1608X90N = smd 0.95 x 1: 1 -0.8,0; 2 0.8,0
0402-1005X55N = smd 0.62 x 0.62: 1 -0.45,0; 2 0.45,0
SMA_DO214AC = smd 1.7 x 1.7: A -1.7,0; C 1.7,0
FD-1-1.5 = smd 1.016 x 1.016: P$1 0,0
SCREW2 = drill 1.3 long: GND 1.27,0; V+ -1.27,0
1X02 = drill 1.016 pad 1.88: 1 -1.27,0; 2 1.27,0
1X02' = drill 1.016 long: 1 -1.27,0; 2 1.27,0
MKRBOARD-SMD-PIN = smd 1 x 5 bottom: 0 42.455,3.61; 1 44.995,3.61; 2 47.535,3.61; 3 50.075,3.61; 4 52.615,3.61; 5 55.155,3.61; 5V 22.135,23.93; 6 55.155,23.93; 7 52.615,23.93; 8 50.075,23.93; 9 47.535,23.93; 10 44.995,23.93; 11 42.455,23.93; 12 39.915,23.93; 13 37.375,23.93; 14 34.835,23.93; A1 27.215,3.61; A2 29.755,3.61; A3 32.295,3.61; A4 34.835,3.61; A5 37.375,3.61; A6 39.915,3.61; AREF 22.135,3.61; DAC0/A0 24.675,3.61; GND 29.755,23.93; RST 32.295,23.93; VCC 27.215,23.93; VIN 24.675,23.93 | hole 2.25: 59.25,3.52; 59.25,24.02; 2.25,3.52; 2.25,24.02
PPTC-1210 = smd 1 x 2.5: P$1 -1.5,0; P$2 1.5,0
TP-1.27MM = smd 1.27 x 1.27 bottom: X 0,0
SOT-23 = smd 0.787 x 0.889: 1 -0.025,1.016; 2 0.94,-1.016; 3 -0.991,-1.016

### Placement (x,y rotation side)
32  39.37,17.65 180 top
70  46.99,6.22 180 top
C1  58.93,20.57 0 top
C2  58.93,18.8 0 top
C3  58.93,8.79 0 top
C4  58.93,6.93 0 top
C5  9.47,20.85 270 top
C6  9.47,16.76 270 top
C7  9.47,12.17 90 top
C8  9.47,8.35 90 top
C9  30.8,16.2 90 bottom
C10  23.3,16.2 90 bottom
C11  38.3,16.2 90 bottom
C12  46,16.2 90 bottom
C13  23.3,11.85 90 bottom
C14  30.8,11.85 90 bottom
C15  38.3,11.85 90 bottom
C16  46,11.85 90 bottom
D1  3.73,19.28 180 bottom
DL1  12.7,25.27 180 top
DL2  16.51,25.27 180 top
DL3  20.32,25.27 180 top
DL4  24.13,25.27 180 top
DL5  27.94,25.27 180 top
DL6  31.75,25.27 180 top
DL7  35.56,25.27 180 top
DL8  39.37,25.27 180 top
DL9  43.18,25.27 180 top
DL10  46.99,25.27 180 top
DL11  50.8,25.27 180 top
DL12  54.61,25.27 180 top
DL13  12.7,21.46 180 top
DL14  16.51,21.46 180 top
DL15  20.32,21.46 180 top
DL16  24.13,21.46 180 top
DL17  27.94,21.46 180 top
DL18  31.75,21.46 180 top
DL19  35.56,21.46 180 top
DL20  39.37,21.46 180 top
DL21  43.18,21.46 180 top
DL22  46.99,21.46 180 top
DL23  50.8,21.46 180 top
DL24  54.61,21.46 180 top
DL25  12.7,17.65 180 top
DL26  16.51,17.65 180 top
DL28  24.13,17.65 180 top
DL29  27.94,17.65 180 top
DL30  31.75,17.65 180 top
DL31  35.56,17.65 180 top
DL33  43.18,17.65 180 top
DL34  46.99,17.65 180 top
DL35  50.8,17.65 180 top
DL36  54.61,17.65 180 top
DL37  12.7,13.84 180 top
DL38  16.51,13.84 180 top
DL39  20.32,13.84 180 top
DL40  24.13,13.84 180 top
DL41  27.94,13.84 180 top
DL42  31.75,13.84 180 top
DL43  35.56,13.84 180 top
DL44  39.37,13.84 180 top
DL45  43.18,13.84 180 top
DL46  46.99,13.84 180 top
DL47  50.8,13.84 180 top
DL48  54.61,13.84 180 top
DL49  12.7,10.03 180 top
DL50  16.51,10.03 180 top
DL51  20.32,10.03 180 top
DL52  24.13,10.03 180 top
DL53  27.94,10.03 180 top
DL54  31.75,10.03 180 top
DL55  35.56,10.03 180 top
DL56  39.37,10.03 180 top
DL57  43.18,10.03 180 top
DL58  46.99,10.03 180 top
DL59  50.8,10.03 180 top
DL60  54.61,10.03 180 top
DL61  12.7,6.22 180 top
DL62  16.51,6.22 180 top
DL63  20.32,6.22 180 top
DL64  24.13,6.22 180 top
DL65  27.94,6.22 180 top
DL66  31.75,6.22 180 top
DL67  35.56,6.22 180 top
DL68  39.37,6.22 180 top
DL69  43.18,6.22 180 top
DL71  50.8,6.22 180 top
DL72  54.61,6.22 180 top
DL73  12.7,2.41 180 top
DL74  16.51,2.41 180 top
DL75  20.32,2.41 180 top
DL76  24.13,2.41 180 top
DL77  27.94,2.41 180 top
DL78  31.75,2.41 180 top
DL79  35.56,2.41 180 top
DL80  39.37,2.41 180 top
DL81  43.18,2.41 180 top
DL82  46.99,2.41 180 top
DL83  50.8,2.41 180 top
DL84  54.61,2.41 180 top
FD1  58.2,1.4 0 bottom
FD2  3.48,26.11 0 top
FD3  3.5,26.1 0 bottom
FD4  58.2,1.4 0 top
FRAME1  0,-1.27 0 top
J1  3.43,14.22 270 top
JANALOG  not placed on the board
JDIGITAL  not placed on the board
JP1  59.18,13.84 270 top
JP2  [1X02']  6.3,3.3 270 top
MKR1  0,0 0 top
PTC  4.06,8.94 0 top
R1  8.05,21.43 90 top
TP1  59.18,17.02 0 top
TP2  59.18,10.67 0 top
TR1  6.6,24.13 90 top
U$29  20.32,17.65 180 top

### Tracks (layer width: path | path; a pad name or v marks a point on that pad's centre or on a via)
+5V  (via drill 0.35)
  Top 0.406: v6.29,26.62 6.35,26.56
  Bottom 0.203: v6.29,26.62 6.29,26.67
  Bottom 1.016: MKR1.5V 22.14,26.63 21.59,26.67 6.29,26.67 5.33,26.67
  other vias: 7.72,26.62 8.43,26.62 5.58,26.62 7.01,26.62
  pour Top (isolate 0.025, rank 5): 4.57,27.43 4.57,25.15 6.22,25.15 6.73,24.64 8.13,24.64 10.92,27.43
  pour Top (no thermals): 4.65,27.18 10.41,27.18 9.4,26.16 4.65,26.16
CKI_ROW1  (via drill 0.35)
  Top 0.305: DL13.5_CKI v11,21.46 | DL12.2_CKO v56.46,25.27
  Route2 0.152: v56.46,25.27 55.37,25.27 13.87,25.27 11.79,23.19 11.79,22 11.25,21.46 v11,21.46
CKI_ROW2  (via drill 0.35)
  Top 0.305: DL25.5_CKI v11,17.65 | DL24.2_CKO v56.46,21.46
  Route2 0.152: v56.46,21.46 13.87,21.46 11.81,19.41 11.81,18.21 11.25,17.65 v11,17.65
CKI_ROW3  (via drill 0.35)
  Top 0.305: v56.46,17.65 DL36.2_CKO | DL37.5_CKI v11,13.84
  Route2 0.152: v56.46,17.65 13.87,17.65 11.79,15.57 11.79,14.38 11.25,13.84 v11,13.84
CKI_ROW4  (via drill 0.35)
  Top 0.305: DL48.2_CKO v56.46,13.84 | DL49.5_CKI v11,10.03
  Route2 0.152: v11,10.03 11.25,10.03 11.79,10.57 11.79,11.74 13.87,13.84 v56.46,13.84
CKI_ROW5  (via drill 0.35)
  Top 0.305: DL61.5_CKI v11,6.22 | DL60.2_CKO v56.46,10.03
  Route2 0.152: v11,6.22 11.23,6.22 11.74,6.73 11.74,7.89 13.87,10.03 v56.46,10.03
CKI_ROW6  (via drill 0.35)
  Top 0.305: DL73.5_CKI v11,2.41 | v56.46,6.22 DL72.2_CKO
  Route2 0.152: v11,2.41 11.25,2.41 11.76,2.92 11.76,4.04 13.87,6.22 55.27,6.22 v56.46,6.22
CKO  (via drill 0.35)
  Top 0.305: DL84.2_CKO v56.46,2.41
  Route15 0.152: v56.46,2.41 56.47,2.41 57,2.94 57,5.41 57.45,5.87 57.45,11.68 58.34,12.57 JP1.2
  Bottom 0.152: TP2.X JP1.2
CKO0
  Top 0.305: DL1.2_CKO DL2.5_CKI
DL27
  Top 0.305: U$29.2_CKO DL28.5_CKI
GND  (via drill 0.35)
  Top 0.152: 23.08,24.4 DL4.6_GND | 30.7,24.4 DL6.6_GND | 38.32,24.4 DL8.6_GND | 45.94,24.4 DL10.6_GND | 53.56,24.4 DL12.6_GND | 45.95,5.36 45.95,5.33 | 34.51,1.54 DL79.6_GND | 11.65,1.54 DL73.6_GND | 53.56,1.54 DL84.6_GND | 30.7,5.35 DL66.6_GND | 38.32,5.35 DL68.6_GND | 11.64,12.96 11.64,12.95 | 15.45,12.96 15.45,12.95 | 19.26,12.96 19.26,12.95 | 23.07,12.96 23.07,12.95 | 26.88,12.96 26.88,12.95 | 30.69,12.96 30.69,12.95 | 34.5,12.96 34.5,12.95 | 38.31,12.96 38.31,12.95 | 42.13,12.97 DL45.6_GND | 45.94,12.97 DL46.6_GND | 49.74,12.96 49.74,12.95 | 53.55,12.96 53.55,12.95 | 15.45,16.77 15.45,16.76 | 19.26,16.77 19.26,16.76 | 23.07,16.77 23.07,16.76 | 34.5,16.77 34.5,16.76 | 42.13,16.78 DL33.6_GND | 45.93,16.77 45.93,16.76 | 49.74,16.77 49.74,16.76 | 11.65,20.59 DL13.6_GND | R1.1 v8.05,20.07 | DL1.GNDPAD 12.7,25.68 | DL68.GNDPAD v39.37,7.7
  Top 0.254: DL8.GNDPAD v39.37,26.92 | DL7.GNDPAD v35.56,26.92 | DL6.GNDPAD v31.75,26.92 | DL5.GNDPAD v27.94,26.92
  Top 0.305: DL12.GNDPAD v54.61,26.92 | DL11.GNDPAD v50.8,26.92 | DL10.GNDPAD v46.99,26.92 | DL9.GNDPAD v43.18,26.92 | DL13.GNDPAD v12.7,22.94 | DL14.GNDPAD v16.51,22.94 | DL15.GNDPAD v20.32,22.94 | DL16.GNDPAD 24.13,22.66 23.75,23.04 v23.7,23.04 | DL17.GNDPAD 27.94,22.78 v28.17,23.04 | DL18.GNDPAD 31.75,22.66 v31.34,23.04 | DL19.GNDPAD 35.56,22.78 v35.79,23.04 | v38.91,23.04 39.37,22.61 DL20.GNDPAD | DL21.GNDPAD 43.18,22.78 v43.41,23.04 | v46.58,23.04 46.99,22.66 DL22.GNDPAD | DL23.GNDPAD 50.8,22.78 v51.03,23.04 | DL25.GNDPAD v12.7,19.13 | DL26.GNDPAD v16.51,19.13 | U$29.GNDPAD v20.32,19.13 | DL28.GNDPAD v24.13,19.13 | DL29.GNDPAD v27.94,19.13 | DL30.GNDPAD v31.75,19.13 | DL31.GNDPAD v35.56,19.13 | 32.GNDPAD v39.37,19.13 | DL33.GNDPAD v43.18,19.13 | DL34.GNDPAD v46.99,19.13 | DL35.GNDPAD v50.8,19.13 | DL36.GNDPAD v54.61,19.13 | DL37.GNDPAD v12.7,15.32 | DL38.GNDPAD v16.51,15.32 | DL39.GNDPAD v20.32,15.32 | DL40.GNDPAD v24.13,15.32 | DL41.GNDPAD v27.94,15.32 | DL42.GNDPAD v31.75,15.32 | DL44.GNDPAD v39.37,15.32 | DL45.GNDPAD v43.18,15.32 | DL46.GNDPAD v46.99,15.32 | DL47.GNDPAD v50.8,15.32 | DL48.GNDPAD v54.61,15.32 | DL43.GNDPAD v35.56,15.32 | DL49.GNDPAD v12.7,11.51 | DL50.GNDPAD v16.51,11.51 | DL53.GNDPAD v27.94,11.51 | DL54.GNDPAD v31.75,11.51 | DL55.GNDPAD v35.56,11.51 | DL56.GNDPAD v39.37,11.51 | DL57.GNDPAD v43.18,11.51 | DL58.GNDPAD v46.99,11.51 | DL59.GNDPAD v50.8,11.51 | DL60.GNDPAD v54.61,11.51 | DL61.GNDPAD v12.7,7.7 | DL62.GNDPAD v16.51,7.7 | DL63.GNDPAD v20.32,7.7 | DL64.GNDPAD v24.13,7.7 | DL65.GNDPAD v27.94,7.7 | DL66.GNDPAD v31.75,7.7 | DL67.GNDPAD v35.56,7.7 | DL69.GNDPAD v43.18,7.7 | 70.GNDPAD v46.99,7.7 | DL71.GNDPAD v50.8,7.7 | DL72.GNDPAD v54.61,7.7
  Top 0.305: v12.7,3.89 DL73.GNDPAD | DL74.GNDPAD v16.51,3.89 | DL75.GNDPAD v20.32,3.89 | DL76.GNDPAD 24.13,3.56 v23.67,3.99 | DL77.GNDPAD 27.94,3.73 v28.17,3.99 | DL79.GNDPAD 35.56,3.73 v35.79,3.99 | DL80.GNDPAD 39.37,3.58 v38.94,3.99 | DL81.GNDPAD 43.18,3.73 v43.41,3.99 | DL82.GNDPAD 46.99,3.61 v46.58,3.99 | DL83.GNDPAD 50.8,3.73 v51.03,3.99 | DL84.GNDPAD 54.61,3.56 v54.15,3.99 | v54.2,23.04 54.3,23.04 54.61,22.73 DL24.GNDPAD | DL51.GNDPAD v20.32,11.51 | DL52.GNDPAD v24.13,11.51 | DL83.6_GND 49.75,0.81 49.76,0.8 v49.76,0.61 | DL13.6_GND 11.01,20.58 v11,20.57 | DL25.6_GND 11.84,16.76 v11,16.76 | DL78.GNDPAD 31.75,3.89 30.9,4.74
  Top 0.356: 12.7,25.68 12.7,26.67 13.08,27.05 16.51,27.05 | 16.51,27.05 20.32,27.05 | DL2.GNDPAD 16.51,27.05 | DL3.GNDPAD 20.32,27.05 | 20.32,27.05 23.37,27.05 | 23.37,27.05 24,27.05 v24.13,26.92 DL4.GNDPAD | v23.37,26.92 23.37,27.05 | v11,16.76 10.2,15.96 C6.2
  Top 0.406: DL84.6_GND 53.57,1.52 v53.57,0.61 | DL73.6_GND 11.64,1.52 v11,1.52 | DL61.6_GND 11.64,5.33 v11,5.33 | 45.95,5.33 70.6_GND 46.15,5.33 v46.15,4.75 | DL60.6_GND 53.55,9.14 v52.7,9.14 | DL59.6_GND 49.74,9.14 v48.9,9.14 | DL58.6_GND 45.93,9.14 v45.09,9.14 | DL57.6_GND 42.12,9.14 v41.27,9.14 | DL56.6_GND 38.31,9.14 v37.47,9.14 | DL55.6_GND 34.5,9.14 v33.66,9.14 | DL54.6_GND 30.69,9.14 v29.84,9.14 | DL53.6_GND 26.88,9.14 v26.04,9.14 | DL52.6_GND 23.07,9.14 v22.23,9.14 | DL51.6_GND 19.26,9.14 v18.41,9.14 | DL50.6_GND 15.45,9.14 v14.61,9.14 | DL49.6_GND 11.64,9.14 v11,9.14 9.67,9.14 C8.2 | DL48.6_GND 53.55,12.95 v52.7,12.95 | DL47.6_GND 49.74,12.95 v48.9,12.95 | DL46.6_GND 45.93,12.95 v45.09,12.95 | DL45.6_GND 42.12,12.95 v41.27,12.95 | DL44.6_GND 38.31,12.95 v37.47,12.95 | DL43.6_GND 34.5,12.95 v33.66,12.95 | DL42.6_GND 30.69,12.95 v29.84,12.95 | DL41.6_GND 26.88,12.95 v26.04,12.95 | DL40.6_GND 23.07,12.95 v22.23,12.95 | DL39.6_GND 19.26,12.95 v18.41,12.95 | DL38.6_GND 15.45,12.95 v14.61,12.95 | DL37.6_GND 11.64,12.95 v11,12.95 9.49,12.95 C7.2 | DL36.6_GND 53.55,16.76 v52.7,16.76 | DL35.6_GND 49.74,16.76 v48.9,16.76 | DL34.6_GND 45.93,16.76 v45.09,16.76 | DL33.6_GND 42.12,16.76 v41.27,16.76 | 32.6_GND 38.31,16.76 v37.47,16.76 | DL31.6_GND 34.5,16.76 v33.66,16.76 | DL30.6_GND 30.69,16.76 v29.84,16.76 | DL29.6_GND 26.88,16.76 v26.04,16.76 | DL28.6_GND 23.07,16.76 v22.23,16.76 | U$29.6_GND 19.26,16.76 v18.41,16.76 | DL26.6_GND 15.45,16.76 v14.61,16.76 | DL14.6_GND 14.62,20.56 v14.61,20.6 | DL15.6_GND 18.43,20.56 v18.41,20.6 | DL16.6_GND v22.24,20.56 v22.23,20.57 | DL17.6_GND v26.05,20.56 v26.04,20.57 | DL18.6_GND 29.86,20.56 v29.84,20.57
  Top 0.406: DL19.6_GND v33.67,20.56 v33.66,20.57 | DL20.6_GND v37.48,20.56 v37.47,20.57 | DL21.6_GND 41.29,20.56 v41.27,20.57 | DL22.6_GND v45.1,20.56 v45.09,20.57 | DL23.6_GND 49.74,20.57 v48.9,20.57 | DL24.6_GND 53.55,20.57 v52.7,20.57 | DL1.6_GND 11.64,24.38 v11,24.38 | v45.95,0.61 DL82.6_GND | v42.14,0.61 DL81.6_GND | v38.33,0.61 DL80.6_GND | v34.52,0.61 34.52,1.53 34.51,1.54 | v23.09,0.61 DL76.6_GND | v19.28,0.61 DL75.6_GND | v15.47,0.61 DL74.6_GND | v26.9,0.61 26.89,0.67 DL77.6_GND | DL62.6_GND 14.72,5.32 v14.63,5.41 | DL68.6_GND v38.52,4.62 v38.51,4.62 | DL66.6_GND 30.9,4.74 v30.89,4.75 | DL64.6_GND 23.28,4.75 v23.09,4.75 | DL63.6_GND 18.48,5.32 v18.41,5.38 | v26.04,5.38 26.1,5.32 DL65.6_GND | v33.68,5.38 33.74,5.32 DL67.6_GND | DL69.6_GND 41.36,5.32 v41.3,5.38 | v48.9,5.38 48.96,5.32 DL71.6_GND | DL4.6_GND 23.28,23.91 v23.27,23.9 | v30.69,23.82 v30.7,23.84 DL6.6_GND | DL8.6_GND 38.32,24.12 38.42,23.86 v38.41,23.85 | v46.15,23.82 v46.14,23.84 DL10.6_GND | v53.75,23.77 53.76,23.79 DL12.6_GND | DL72.6_GND 53.75,5.33 v53.75,4.75 | C5.2 10.47,20.05 v11,20.57 | DL2.6_GND 15.65,24.38 v14.61,24.38 | DL3.6_GND 19.46,24.38 v18.44,24.38 | DL5.6_GND 27.08,24.38 v26.06,24.38 | DL7.6_GND 34.7,24.38 v33.68,24.38 | DL9.6_GND 42.32,24.38 v41.27,24.38 | DL11.6_GND 49.94,24.38 v48.92,24.38 | DL78.6_GND 30.7,0.54 30.73,0.51 v30.73,0.6
  Top 0.813: v60.7,18.8 C2.2 | v60.7,6.93 C4.2 | v60.7,8.73 60.74,8.78 60.77,8.79 C3.2 | v60.7,20.57 C1.2
  Bottom 0.406: v30.73,0.6 31.15,0.6 31.24,0.51
  pour Bottom (rank 6, no thermals): 0,0 0,27.43 61.47,27.43 61.47,0
  pour Route15: 0,0 0,27.5 61.4,27.5 61.4,0
LEDCKI  (via drill 0.35)
  Top 0.305: v11,25.27 DL1.5_CKI
  Bottom 0.152: MKR1.A4 34.84,7.96 34.19,8.61 9.47,8.61 8.89,9.19 8.89,18.8 9.2,19.1 9.2,23.47 v11,25.27
LEDSDI  (via drill 0.35)
  Top 0.152: v9.53,24.8 10.93,26.2 DL1.4_SDI
  Bottom 0.152: MKR1.A3 32.3,7.99 31.98,8.31 9.27,8.31 8.49,9.09 8.49,19.13 8.77,19.41 8.77,24.06 9.51,24.8 v9.53,24.8
N$1
  Top 0.305: DL2.3_SDO DL3.4_SDI
N$2
  Top 0.305: DL2.2_CKO DL3.5_CKI
N$3
  Top 0.305: DL3.3_SDO DL4.4_SDI
N$4
  Top 0.305: DL3.2_CKO DL4.5_CKI
N$5
  Top 0.305: DL4.3_SDO DL5.4_SDI
N$6
  Top 0.305: DL4.2_CKO DL5.5_CKI
N$7
  Top 0.305: DL5.3_SDO DL6.4_SDI
N$8
  Top 0.305: DL5.2_CKO DL6.5_CKI
N$9
  Top 0.305: DL6.3_SDO DL7.4_SDI
N$10
  Top 0.305: DL6.2_CKO DL7.5_CKI
N$11
  Top 0.305: DL7.3_SDO DL8.4_SDI
N$12
  Top 0.305: DL7.2_CKO DL8.5_CKI
N$13
  Top 0.305: DL8.3_SDO DL9.4_SDI
N$14
  Top 0.305: DL8.2_CKO DL9.5_CKI
N$15
  Top 0.305: DL9.3_SDO DL10.4_SDI
N$16
  Top 0.305: DL9.2_CKO DL10.5_CKI
N$17
  Top 0.305: DL10.3_SDO DL11.4_SDI
N$18
  Top 0.305: DL10.2_CKO DL11.5_CKI
N$19
  Top 0.305: DL11.3_SDO DL12.4_SDI
N$20
  Top 0.305: DL11.2_CKO DL12.5_CKI
N$21
  Top 0.305: DL13.3_SDO DL14.4_SDI
N$22
  Top 0.305: DL13.2_CKO DL14.5_CKI
N$23
  Top 0.305: DL14.3_SDO DL15.4_SDI
N$24
  Top 0.305: DL14.2_CKO DL15.5_CKI
N$25
  Top 0.305: DL15.3_SDO DL16.4_SDI
N$26
  Top 0.305: DL15.2_CKO DL16.5_CKI
N$27
  Top 0.305: DL16.3_SDO DL17.4_SDI
N$28
  Top 0.305: DL16.2_CKO DL17.5_CKI
N$29
  Top 0.305: DL17.3_SDO DL18.4_SDI
N$30
  Top 0.305: DL17.2_CKO DL18.5_CKI
N$31
  Top 0.305: DL18.3_SDO DL19.4_SDI
N$32
  Top 0.305: DL18.2_CKO DL19.5_CKI
N$33
  Top 0.305: DL19.3_SDO DL20.4_SDI
N$34
  Top 0.305: DL19.2_CKO DL20.5_CKI
N$35
  Top 0.305: DL20.3_SDO DL21.4_SDI
N$36
  Top 0.305: DL20.2_CKO DL21.5_CKI
N$37
  Top 0.152: DL21.3_SDO DL22.4_SDI
N$38
  Top 0.152: DL21.2_CKO DL22.5_CKI
N$39
  Top 0.305: DL22.3_SDO DL23.4_SDI
N$40
  Top 0.305: DL22.2_CKO DL23.5_CKI
N$41
  Top 0.305: DL23.3_SDO DL24.4_SDI
N$42
  Top 0.305: DL23.2_CKO DL24.5_CKI
N$43
  Top 0.305: DL25.3_SDO DL26.4_SDI
N$44
  Top 0.305: DL25.2_CKO DL26.5_CKI
N$45
  Top 0.305: DL26.3_SDO U$29.4_SDI
N$46
  Top 0.305: DL26.2_CKO U$29.5_CKI
N$47
  Top 0.305: U$29.3_SDO DL28.4_SDI
N$49
  Top 0.305: DL28.3_SDO DL29.4_SDI
N$50
  Top 0.305: DL28.2_CKO DL29.5_CKI
N$51
  Top 0.305: DL29.3_SDO DL30.4_SDI
N$52
  Top 0.305: DL29.2_CKO DL30.5_CKI
N$53
  Top 0.305: DL30.3_SDO DL31.4_SDI
N$54
  Top 0.305: DL30.2_CKO DL31.5_CKI
N$55
  Top 0.305: DL31.3_SDO 32.4_SDI
N$56
  Top 0.305: DL31.2_CKO 32.5_CKI
N$57
  Top 0.305: 32.3_SDO DL33.4_SDI
N$58
  Top 0.305: 32.2_CKO DL33.5_CKI
N$59
  Top 0.305: DL33.3_SDO DL34.4_SDI
N$60
  Top 0.305: DL33.2_CKO DL34.5_CKI
N$61
  Top 0.305: DL34.3_SDO DL35.4_SDI
N$62
  Top 0.305: DL34.2_CKO DL35.5_CKI
N$63
  Top 0.305: DL35.3_SDO DL36.4_SDI
N$64
  Top 0.305: DL35.2_CKO DL36.5_CKI
N$65
  Top 0.305: DL37.3_SDO DL38.4_SDI
N$66
  Top 0.305: DL37.2_CKO DL38.5_CKI
N$67
  Top 0.305: DL38.3_SDO DL39.4_SDI
N$68
  Top 0.305: DL38.2_CKO DL39.5_CKI
N$69
  Top 0.305: DL39.3_SDO DL40.4_SDI
N$70
  Top 0.305: DL39.2_CKO DL40.5_CKI
N$71
  Top 0.305: DL40.3_SDO DL41.4_SDI
N$72
  Top 0.305: DL40.2_CKO DL41.5_CKI
N$73
  Top 0.305: DL41.3_SDO DL42.4_SDI
N$74
  Top 0.305: DL41.2_CKO DL42.5_CKI
N$75
  Top 0.305: DL42.3_SDO DL43.4_SDI
N$76
  Top 0.305: DL42.2_CKO DL43.5_CKI
N$77
  Top 0.305: DL43.3_SDO DL44.4_SDI
N$78
  Top 0.305: DL43.2_CKO DL44.5_CKI
N$79
  Top 0.305: DL44.3_SDO DL45.4_SDI
N$80
  Top 0.305: DL44.2_CKO DL45.5_CKI
N$81
  Top 0.305: DL45.3_SDO DL46.4_SDI
N$82
  Top 0.305: DL45.2_CKO DL46.5_CKI
N$83
  Top 0.305: DL46.3_SDO DL47.4_SDI
N$84
  Top 0.305: DL46.2_CKO DL47.5_CKI
N$85
  Top 0.305: DL47.3_SDO DL48.4_SDI
N$86
  Top 0.305: DL47.2_CKO DL48.5_CKI
N$87
  Top 0.305: DL50.3_SDO DL51.4_SDI
N$88
  Top 0.305: DL50.2_CKO DL51.5_CKI
N$89
  Top 0.305: DL51.3_SDO DL52.4_SDI
N$90
  Top 0.305: DL51.2_CKO DL52.5_CKI
N$91
  Top 0.305: DL52.3_SDO DL53.4_SDI
N$92
  Top 0.305: DL52.2_CKO DL53.5_CKI
N$93
  Top 0.305: DL53.3_SDO DL54.4_SDI
N$94
  Top 0.305: DL53.2_CKO DL54.5_CKI
N$95
  Top 0.305: DL54.3_SDO DL55.4_SDI
N$96
  Top 0.305: DL54.2_CKO DL55.5_CKI
N$97
  Top 0.305: DL55.3_SDO DL56.4_SDI
N$98
  Top 0.305: DL55.2_CKO DL56.5_CKI
N$99
  Top 0.305: DL56.3_SDO DL57.4_SDI
N$100
  Top 0.305: DL56.2_CKO DL57.5_CKI
N$101
  Top 0.305: DL57.3_SDO DL58.4_SDI
N$102
  Top 0.305: DL57.2_CKO DL58.5_CKI
N$103
  Top 0.305: DL58.3_SDO DL59.4_SDI
N$104
  Top 0.305: DL58.2_CKO DL59.5_CKI
N$105
  Top 0.305: DL59.3_SDO DL60.4_SDI
N$106
  Top 0.305: DL59.2_CKO DL60.5_CKI
N$107
  Top 0.305: DL49.3_SDO DL50.4_SDI
N$108
  Top 0.305: DL49.2_CKO 13.97,10.03 14.22,10.03 DL50.5_CKI
N$109
  Top 0.305: DL61.3_SDO DL62.4_SDI
N$110
  Top 0.305: DL61.2_CKO DL62.5_CKI
N$111
  Top 0.305: DL62.3_SDO DL63.4_SDI
N$112
  Top 0.305: DL62.2_CKO DL63.5_CKI
N$113
  Top 0.305: DL73.3_SDO DL74.4_SDI
N$114
  Top 0.305: DL73.2_CKO DL74.5_CKI
N$115
  Top 0.305: DL74.3_SDO DL75.4_SDI
N$116
  Top 0.305: DL74.2_CKO DL75.5_CKI
N$117
  Top 0.305: DL63.3_SDO DL64.4_SDI
N$118
  Top 0.305: DL63.2_CKO DL64.5_CKI
N$119
  Top 0.305: DL75.3_SDO DL76.4_SDI
N$120
  Top 0.305: DL75.2_CKO DL76.5_CKI
N$121
  Top 0.305: DL64.3_SDO DL65.4_SDI
N$122
  Top 0.305: DL64.2_CKO DL65.5_CKI
N$123
  Top 0.305: DL76.3_SDO DL77.4_SDI
N$124
  Top 0.305: DL76.2_CKO DL77.5_CKI
N$125
  Top 0.305: DL65.3_SDO DL66.4_SDI
N$126
  Top 0.305: DL65.2_CKO DL66.5_CKI
N$127
  Top 0.305: DL77.3_SDO DL78.4_SDI
N$128
  Top 0.305: DL77.2_CKO DL78.5_CKI
N$129
  Top 0.305: DL66.3_SDO DL67.4_SDI
N$130
  Top 0.305: DL66.2_CKO DL67.5_CKI
N$131
  Top 0.305: DL78.3_SDO DL79.4_SDI
N$132
  Top 0.305: DL78.2_CKO DL79.5_CKI
N$133
  Top 0.305: DL67.3_SDO DL68.4_SDI
N$134
  Top 0.305: DL67.2_CKO DL68.5_CKI
N$135
  Top 0.305: DL79.3_SDO DL80.4_SDI
N$136
  Top 0.305: DL79.2_CKO DL80.5_CKI
N$137
  Top 0.305: DL68.3_SDO DL69.4_SDI
N$138
  Top 0.305: DL68.2_CKO DL69.5_CKI
N$139
  Top 0.305: DL80.3_SDO DL81.4_SDI
N$140
  Top 0.305: DL80.2_CKO DL81.5_CKI
N$141
  Top 0.305: DL69.3_SDO 70.4_SDI
N$142
  Top 0.305: DL69.2_CKO 70.5_CKI
N$143
  Top 0.305: DL81.3_SDO DL82.4_SDI
N$144
  Top 0.305: DL81.2_CKO DL82.5_CKI
N$145
  Top 0.305: 70.3_SDO DL71.4_SDI
N$146
  Top 0.305: 70.2_CKO DL71.5_CKI
N$147
  Top 0.305: DL82.3_SDO DL83.4_SDI
N$148
  Top 0.305: DL82.2_CKO DL83.5_CKI
N$149
  Top 0.305: DL71.3_SDO DL72.4_SDI
N$150
  Top 0.305: DL71.2_CKO DL72.5_CKI
N$151
  Top 0.305: DL83.3_SDO DL84.4_SDI
N$152
  Top 0.305: DL83.2_CKO DL84.5_CKI
RESET  (via drill 0.35)
  Top 0.203: v9.66,10.15 8.63,10.15 8.13,9.65 8.13,6.39 JP2.1
  Bottom 0.152: MKR1.RST 32.3,21.77 32.4,21.66 32.4,14.1 32.34,14.04 13.18,14.04 9.66,10.52 v9.66,10.15
SDI_ROW1  (via drill 0.35)
  Top 0.305: DL13.4_SDI 11.85,22.34 v11,22.34 | DL12.3_SDO 56.18,26.15 v56.46,26.15
  Route2 0.152: v56.46,26.15 55.94,25.63 13.44,25.63 11,23.19 v11,22.34
SDI_ROW2  (via drill 0.35)
  Top 0.305: DL24.3_SDO v56.46,22.36 | DL25.4_SDI 11.85,18.53 v11,18.53
  Route2 0.152: v56.46,22.36 55.95,21.84 13.44,21.84 11,19.41 v11,18.53
SDI_ROW3  (via drill 0.35)
  Top 0.305: DL37.4_SDI 11.05,14.72 v11,14.73 | DL36.3_SDO 56.63,18.55 v56.46,18.54
  Route2 0.152: v56.46,18.54 55.96,18.03 55.68,18.03 13.44,18.03 11,15.6 v11,14.73
SDI_ROW4  (via drill 0.35)
  Top 0.305: DL48.3_SDO v56.46,14.74 | DL49.4_SDI 11.85,10.91 v11,10.91
  Route2 0.152: v11,10.91 11,11.77 10.98,11.77 13.44,14.22 55.95,14.22 v56.46,14.74
SDI_ROW5  (via drill 0.35)
  Top 0.305: v11,7.13 10.95,7.1 DL61.4_SDI | DL60.3_SDO 55.47,10.92 v56.46,10.92
  Route2 0.152: v56.46,10.92 55.93,10.39 29.26,10.39 13.44,10.39 11,7.97 v11,7.13
SDI_ROW6  (via drill 0.35)
  Top 0.305: DL73.4_SDI v10.99,3.29 v11,3.29 | DL72.3_SDO 55.47,7.11 v56.46,7.11
  Route2 0.152: v56.46,7.11 55.93,6.58 55.17,6.58 13.44,6.58 11.65,4.72 11,4.06 v11,3.29
SDO  (via drill 0.35)
  Top 0.406: v56.46,3.3 56.57,3.28 DL84.3_SDO
  Route15 0.152: v56.46,3.3 56.46,5.45 57.15,6.1 57.15,14.81 57.45,15.11 JP1.1
  Bottom 0.152: TP1.X JP1.1
SDO0
  Top 0.305: DL1.3_SDO DL2.4_SDI
VCC_LED  (via drill 0.35)
  Top 0.152: 12.72,5.32 12.7,5.3 | 16.53,5.32 16.51,5.3
  Top 0.305: 70.VDDPAD 46.99,5.22
  Top 0.406: v29.85,15.75 29.7,15.75 29.6,15.85
  Bottom 0.406: C10.1 v22.2,15.75 | C9.1 v29.85,15.75 | C11.1 v37.45,15.75 | v37.45,11.65 37.7,11.4 C15.1 | v29.85,11.54 30.04,11.35 30.75,11.35 C14.1 | C13.1 22.45,11.4 v22.2,11.65 | C12.1 v45.1,15.75 | C16.1 45.4,11.4 v45.1,11.7
  other vias: 1.14,10.77 2.16,10.77 3.17,10.77 1.14,7.09 2.16,7.09 3.17,7.11 11.56,0.61 18.41,0.61 22.23,0.61 26.04,0.61 29.84,0.61 33.66,0.61 37.47,0.61 41.27,0.61 45.09,0.61 48.9,0.61 52.7,0.61 56.52,0.61 7.75,16.61 7.75,17.63 7.75,18.65 7.75,11.53 7.75,10.52 7.24,9.5 7.24,8.49 7.24,7.47 41.27,23.22 36.35,23.73 48.92,23.22 26.06,23.22 26.04,4.17 33.55,4.19 41.2,4.19 48.9,4.17
  pour Route2: 0,-0.1 0,27.4 61.4,27.4 61.4,-0.1
  pour Top (isolate 0.025, rank 3): 61.47,0 0,0 0,13.97 4.65,13.97 4.65,24.79 4.55,24.82 6.12,24.82 6.81,24.13 8.13,24.13 11.18,27.18 61.47,27.43
VCC_PTC  (via drill 0.4)
  Top 1.27: v5.43,20.68 5.59,20.53 | 5.59,20.53 5.59,20.83 | v5.43,17.78 5.59,20.53
  Bottom 1.27: v5.43,20.68 D1.C 5.43,17.93 v5.43,17.78
  pour Top (no thermals): 4.62,24.84 4.62,18.31 4.67,7.59 6.05,7.59 6.38,7.92 6.38,24.41 5.94,24.84
VIN  (via drill 0.35)
  Top 0.152: 7.28,21.88 v7.26,21.89
  Top 0.203: 3.02,20.75 1.8,19.61
  Top 0.305: TR1.3 7.62,23.09 8.05,22.67 R1.2 7.28,21.88
  Top 0.61: v9.47,14.48 v7.92,14.48
  Bottom 0.305: v7.26,21.89 7.26,21.77 3.48,21.77 2.72,21.01
  Bottom 0.356: MKR1.VIN
  Bottom 0.6: 10.72,19.41 9.47,18.16
  Bottom 0.61: J1.V+ 4.88,15.49 5.89,14.48 v7.92,14.48 | v9.47,14.48 9.47,18.16 | 10.72,19.41 11.58,19.41 12.13,19.96 13.42,19.96 13.53,19.84 15.83,19.84 15.94,19.96 17.23,19.96 17.34,19.84 19.64,19.84 19.75,19.96 21.01,19.96 21.15,19.82 23.43,19.82 24.64,21.03 24.64,23.89 MKR1.VIN
  other vias: 1.96,21.01
  pour Top (rank 3, no thermals): 0,21.36 3.81,21.36 3.81,16.51 3.84,16.48 3.84,14.5 0.74,14.5 0,15.24
  pour Bottom (rank 5, no thermals): 0.25,21.34 3.81,21.34 3.81,14.48 0.51,14.48 0.25,14.73

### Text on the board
tPlace: DO | + | - | CO
bPlace: DO | CO

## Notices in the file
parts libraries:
Arduino-utility: Copyright (c) 2016-2017 Arduino LLC. All right reserved.
